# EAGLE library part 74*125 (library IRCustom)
Quad bus BUFFER, 3-state
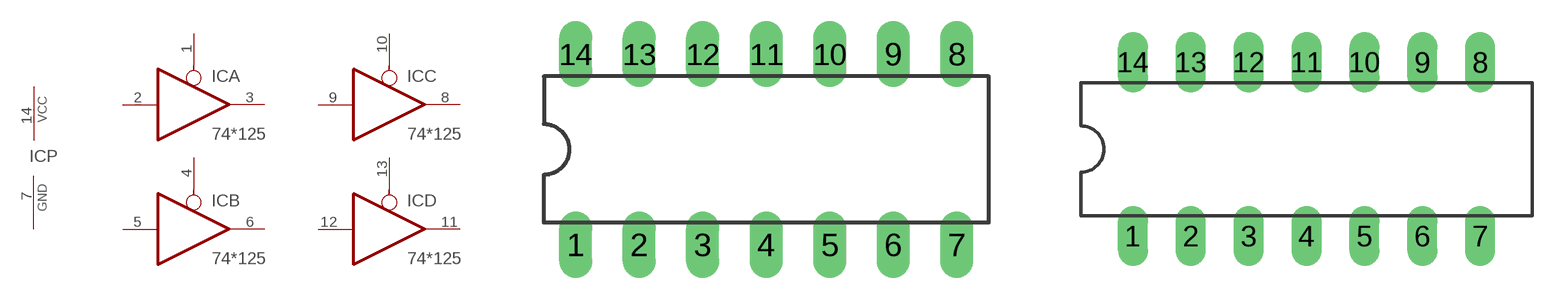
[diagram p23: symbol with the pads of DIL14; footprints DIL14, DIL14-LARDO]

Designator prefix IC; gates A=74125 B=74125 C=74125 D=74125 P=PWRN

## 74125N, 74LS125N  [DIL14]
1  A:OE  in
2  A:I  in
3  A:O  hiz
4  B:OE  in
5  B:I  in
6  B:O  hiz
7  P:GND  pwr
8  C:O  hiz
9  C:I  in
10  C:OE  in
11  D:O  hiz
12  D:I  in
13  D:OE  in
14  P:VCC  pwr

## 74125N-LARDO  [DIL14-LARDO]
Pads as for DIL14

## Footprint DIL14 (pad centres in mm)
Dual In Line Package
drill 0.813 long: 1 -7.62,-3.81; 2 -5.08,-3.81; 3 -2.54,-3.81; 4 0,-3.81; 5 2.54,-3.81; 6 5.08,-3.81; 7 7.62,-3.81; 8 7.62,3.81; 9 5.08,3.81; 10 2.54,3.81; 11 0,3.81; 12 -2.54,3.81; 13 -5.08,3.81; 14 -7.62,3.81

## Footprint DIL14-LARDO (pad centres in mm)
drill 0.813 long: 1 -7.62,-3.81; 2 -5.08,-3.81; 3 -2.54,-3.81; 4 0,-3.81; 5 2.54,-3.81; 6 5.08,-3.81; 7 7.62,-3.81; 8 7.62,3.81; 9 5.08,3.81; 10 2.54,3.81; 11 0,3.81; 12 -2.54,3.81; 13 -5.08,3.81; 14 -7.62,3.81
